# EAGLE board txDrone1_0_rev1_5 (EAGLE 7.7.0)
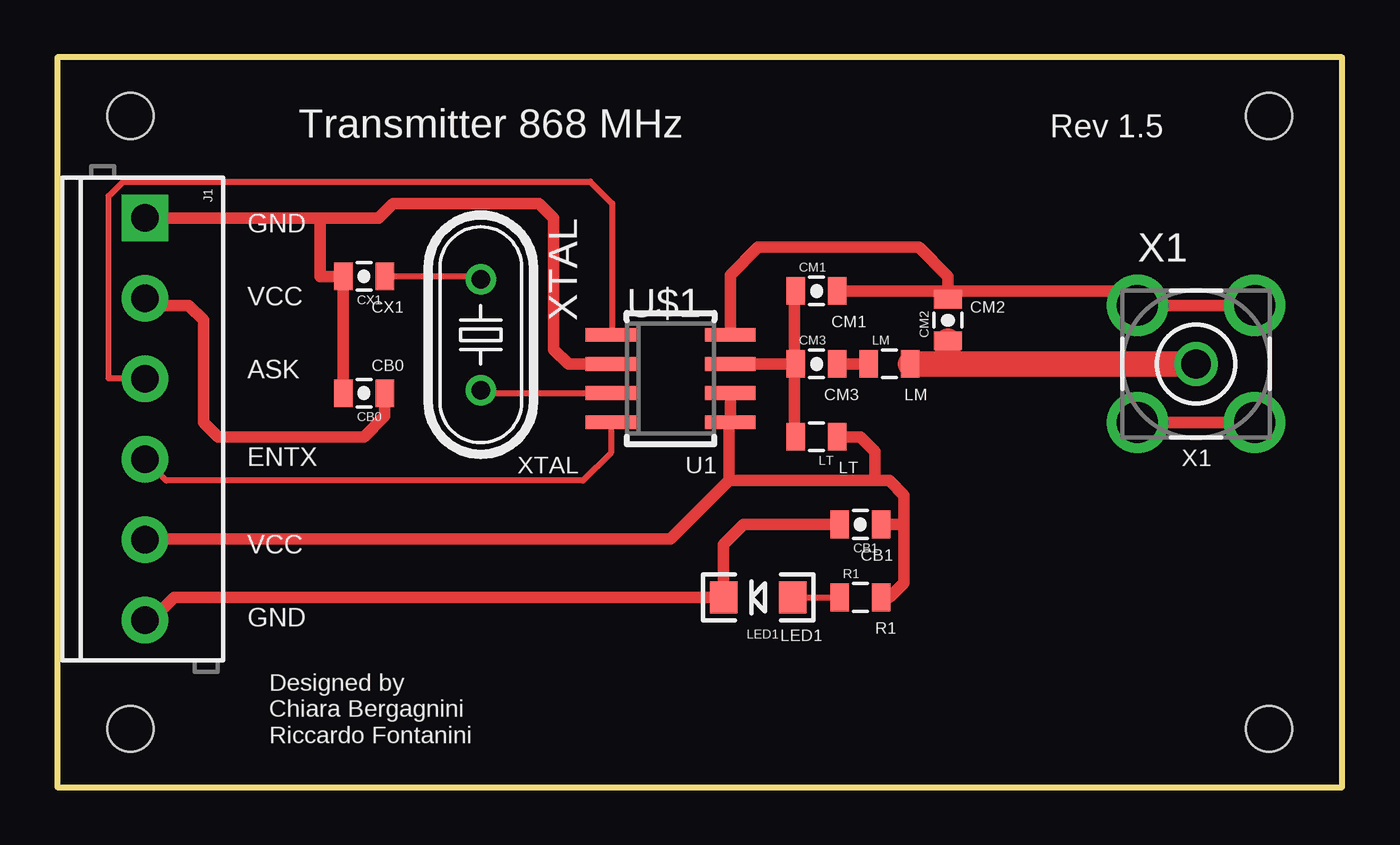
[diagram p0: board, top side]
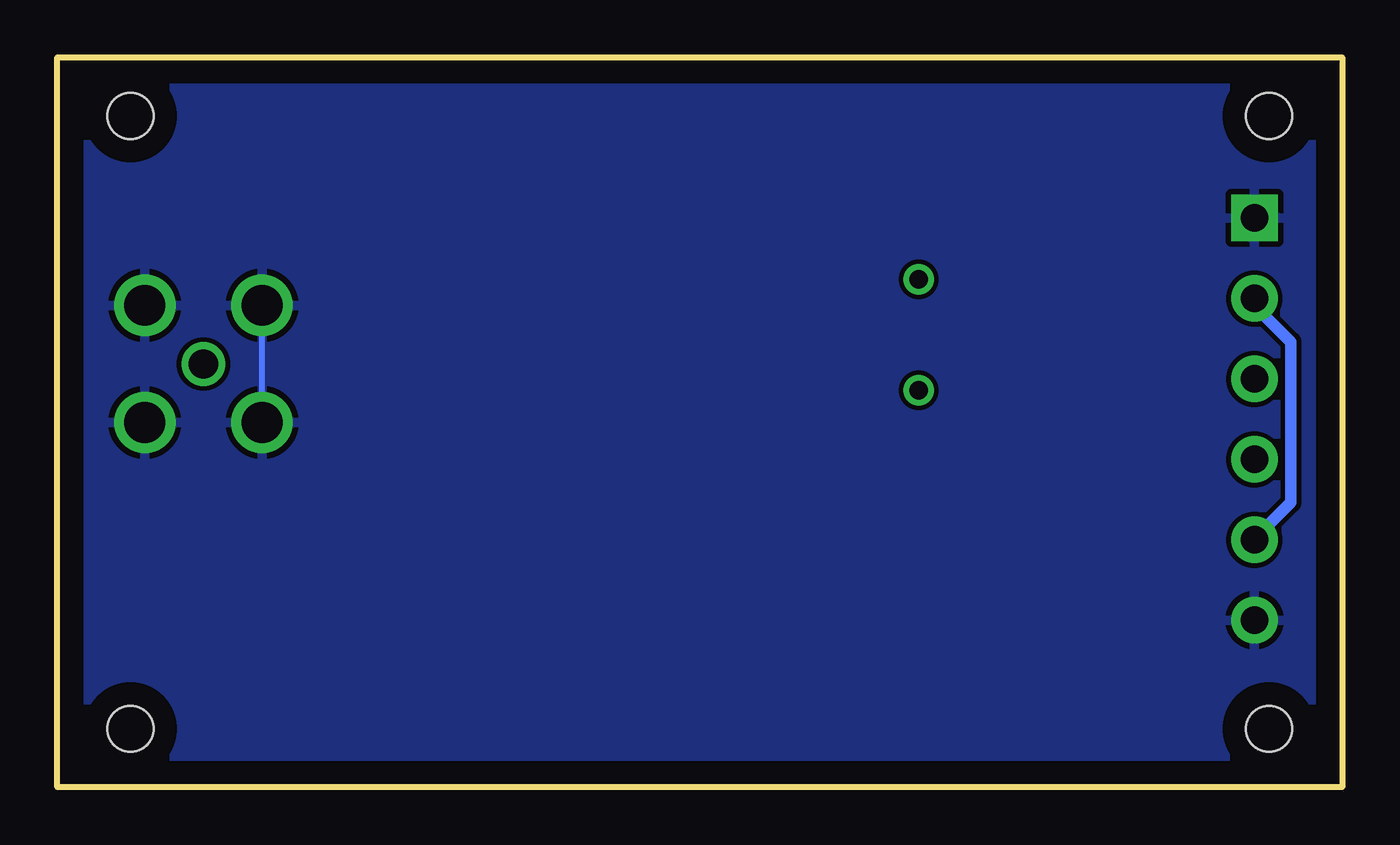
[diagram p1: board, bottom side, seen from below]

Size 55.88 x 31.75 mm. Coordinates in mm from the lower left corner, seen from the top.
Outline: 0,0 55.88,0 55.88,31.75 0,31.75 0,0
Copper layers (1*16): Top 0.035mm / dielectric 1.5mm / Bottom 0.035mm
Design rules "default *": minimum track width 10mil, minimum drill 24mil, track to track 8mil, track to pad 8mil, pad to pad 8mil, via to via 8mil, smd to smd 8mil, copper to edge 40mil, drill to drill 8mil, minimum pad ring 10mil, minimum via ring 8mil, stop-mask expansion 4mil, vias tented up to drill 2mil, thermal gap 10mil
Holes 2 mm at 52.7,2.54 52.7,29.21 3.17,29.21 3.17,2.54

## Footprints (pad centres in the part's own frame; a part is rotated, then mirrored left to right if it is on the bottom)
0805-CAP = smd 0.8 x 1.2: 1 -0.9,0; 2 0.9,0
SCREWTERMINAL-3.5MM-6@1 = drill 1.2 pad 2.032 square: 1 0,0 | drill 1.2 pad 2.032: 2 3.5,0; 3 7,0; 4 10.5,0; 5 14,0; 6 17.5,0
LED-1206 = smd 1.2 x 1.4: A -1.5,0; C 1.5,0
0805 = smd 0.8 x 1.2: 1 -0.9,0; 2 0.9,0
SO08 = smd 0.6 x 2.2: 1 -1.905,-2.6; 2 -0.635,-2.6; 3 0.635,-2.6; 4 1.905,-2.6; 5 1.905,2.6; 6 0.635,2.6; 7 -0.635,2.6; 8 -1.905,2.6
BU-SMA-V = drill 1.27: 1 0,0 | drill 1.778: 2 -2.55,2.55; 3 2.55,2.55; 4 2.55,-2.55; 5 -2.55,-2.55
HC49U-V = drill 0.813: 1 -2.413,0; 2 2.413,0

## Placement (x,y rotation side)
CB0  220nF  [0805-CAP]  13.34,17.14 180 top
CB1  330pF  [0805-CAP]  34.92,11.43 180 top
CM1  1.8pF  [0805-CAP]  33.02,21.59 0 top
CM2  5.6pF  [0805-CAP]  38.73,20.32 90 top
CM3  68pF  [0805-CAP]  33.02,18.41 0 top
CX1  27pF  [0805-CAP]  13.34,22.23 180 top
J1  [SCREWTERMINAL-3.5MM-6@1]  3.81,24.77 270 top
LED1  [LED-1206]  30.48,8.26 180 top
LM  12nH  [0805]  36.2,18.41 0 top
LT  15nH  [0805]  33.02,15.24 180 top
R1  220  [0805]  34.92,8.26 0 top
U$1  TH72032NORMAL  [SO08]  26.67,17.78 270 top
X1  BU-SMA-V  [BU-SMA-V]  49.53,18.41 0 top
XTAL  [HC49U-V]  18.41,19.68 270 top

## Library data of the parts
CB0 CB1 CM1-CM3 CX1 = SparkFun-Capacitors; PROD_ID: CAP-11624
J1 = SparkFun-Connectors
LED1 = SparkFun-LED
LM LT = SparkFun-Passives
R1 = SparkFun-Resistors
U$1 = th72032
X1 = con-coax; OC_FARNELL: unknown; OC_NEWARK: unknown
XTAL = SparkFun-FreqCtrl

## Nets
GND: CB0.2 CB1.2 CM1.2 CM2.2 CX1.2 J1.1 J1.6 LED1.C U$1.2 U$1.8 X1.2 X1.3 X1.4 X1.5
N$1: CM1.1 CM3.1 LT.2 U$1.7
N$2: CM3.2 LM.1
N$3: CM2.1 LM.2 X1.1
N$4: U$1.3 XTAL.2
N$5: CX1.1 XTAL.1
N$6: J1.3 U$1.1
N$7: J1.4 U$1.4
N$8: LED1.A R1.1
VCC: CB0.1 CB1.1 J1.2 J1.5 LT.1 R1.2 U$1.5 U$1.6

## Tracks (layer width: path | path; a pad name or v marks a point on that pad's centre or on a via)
GND
  Top 0.254: X1.5 | X1.4 | X1.3 | X1.2 | U$1.2 23.81,18.41
  Top 0.508: X1.4 X1.5 | X1.2 X1.3 | J1.6 4.09,7.26 5.08,8.26 LED1.C 28.98,10.56 29.84,11.43 CB1.2 | U$1.8 29.27,22.29 30.48,23.5 37.47,23.5 38.73,22.23 38.73,21.59 | 38.73,21.59 CM1.2 | 38.73,21.59 46.35,21.59 X1.2 | CM2.2 38.73,21.59 | CB0.2 CX1.2 11.43,22.23 11.43,24.77 | U$1.2 22.23,18.41 21.59,19.05 21.59,24.77 20.95,25.4 14.61,25.4 13.97,24.77 11.43,24.77 | J1.1 11.43,24.77
  Bottom 0.254: X1.5 X1.2
  pour Bottom: 0.64,0.64 55.24,0.64 55.88,32.38 0.64,31.75
N$1
  Top 0.254: 32.07,15.24 LT.2 | 32.07,21.59 CM1.1 | 32.07,18.41 CM3.1
  Top 0.508: 32.07,18.41 32.07,15.24 | 32.07,18.41 32.07,21.59 | 32.07,18.41 U$1.7
N$2
  Top 0.508: LM.1 CM3.2
N$3
  Top 1.118: LM.2 38.73,18.41 | 38.73,18.41 X1.1 | CM2.1 38.73,18.41
N$4
  Top 0.254: U$1.3 18.41,17.14 XTAL.2
N$5
  Top 0.254: CX1.1 18.41,22.23 XTAL.1
N$6
  Top 0.254: 23.81,19.68 U$1.1 24.13,19.75 24.13,25.4 23.18,26.35 2.86,26.35 2.22,25.72 2.22,17.78 J1.3
N$7
  Top 0.254: U$1.4 24.07,14.54 22.86,13.34 4.74,13.34 J1.4
N$8
  Top 0.254: LED1.A R1.1
VCC
  Top 0.508: J1.5 arc-90 3.84,10.79 26.67,10.79 29.21,13.34 | CB1.1 36.83,11.43 | 36.83,11.43 36.83,8.89 36.2,8.26 R1.2 | U$1.6 U$1.5 29.21,15.81 29.21,13.34 | CB0.1 14.23,16.14 13.34,15.24 6.99,15.24 6.35,15.88 6.35,20.32 5.71,20.95 4.12,20.95 J1.2 | 36.83,11.43 36.83,12.7 36.2,13.34 35.56,13.34 | 35.56,13.34 29.21,13.34 | LT.1 34.92,15.24 35.56,14.61 35.56,13.34
  Bottom 0.254: 3.81,10.79 J1.5 | 3.81,20.95 J1.2
  Bottom 0.508: 3.81,10.79 2.22,12.38 2.22,19.37 3.81,20.95

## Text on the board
tPlace: Transmitter 868 MHz | Rev 1.5 | GND | VCC | CX1 | CM2 | CM1 | ASK | CB0 | CM3 | LM | ENTX | XTAL | U1 | LT | X1 | VCC | CB1 | GND | R1 | LED1 | Designed by / Chiara Bergagnini / Riccardo Fontanini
